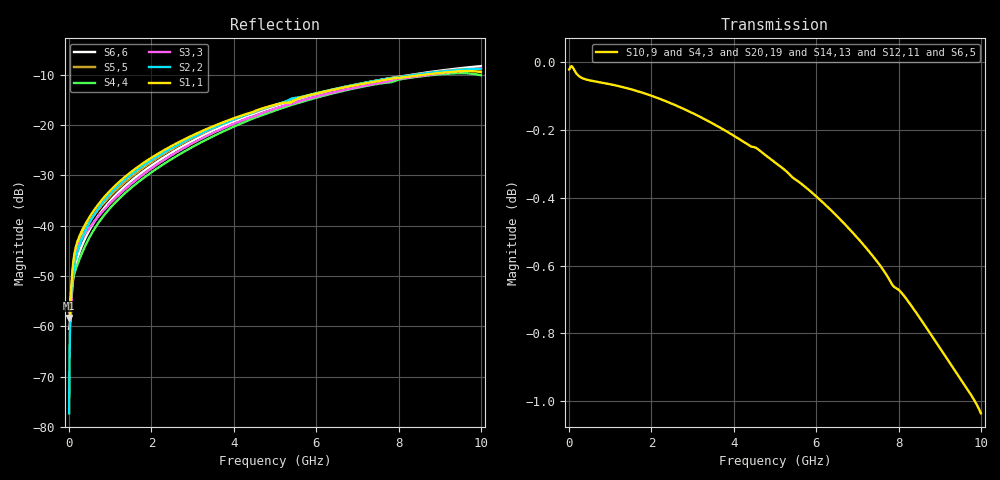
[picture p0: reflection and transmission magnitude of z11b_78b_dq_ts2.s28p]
![Disclaimer] This software code/ model/ data and all associated documentation, comments
!    or other information (collectively "Software") is provided
!    "AS IS" without warranty of any kind. MICRON TECHNOLOGY, INC.
!   ("MTI") EXPRESSLY DISCLAIMS ALL WARRANTIES EXPRESS OR IMPLIED,
!    INCLUDING BUT NOT LIMITED TO, NONINFRINGEMENT OF THIRD PARTY
!   RIGHTS, AND ANY IMPLIED WARRANTIES OF MERCHANTABILITY OR FITNESS
!    FOR ANY PARTICULAR PURPOSE. MTI DOES NOT WARRANT THAT THE
!    SOFTWARE WILL MEET YOUR REQUIREMENTS, OR THAT THE OPERATION OF
!    THE SOFTWARE WILL BE UNINTERRUPTED OR ERROR-FREE. FURTHERMORE,
!    MTI DOES NOT MAKE ANY REPRESENTATIONS REGARDING THE USE OR THE
!    RESULTS OF THE USE OF THE SOFTWARE IN TERMS OF ITS CORRECTNESS,
!    ACCURACY, RELIABILITY, OR OTHERWISE. THE ENTIRE RISK ARISING OUT
!    OF USE OR PERFORMANCE OF THE SOFTWARE REMAINS WITH YOU. IN NO
!    EVENT SHALL MTI, ITS AFFILIATED COMPANIES OR THEIR SUPPLIERS BE
!    LIABLE FOR ANY DIRECT, INDIRECT, CONSEQUENTIAL, INCIDENTAL, OR
!    SPECIAL DAMAGES (INCLUDING, WITHOUT LIMITATION, DAMAGES FOR LOSS
!    OF PROFITS, BUSINESS INTERRUPTION, OR LOSS OF INFORMATION)
!    ARISING OUT OF YOUR USE OF OR INABILITY TO USE THE SOFTWARE,
!    EVEN IF MTI HAS BEEN ADVISED OF THE POSSIBILITY OF SUCH DAMAGES.
!    Because some jurisdictions prohibit the exclusion or limitation
!    of liability for consequential or incidental damages, the above
!    limitation may not apply to you.
!    Copyright 2019 Micron Technology, Inc. All rights reserved.
! Single-ended  S-parameters
!NUMBER OF PORTS = 28
!  PORT#  PORT_NAME  NET_NAME
! PORT1:  DM#-BGA.A7 DM#
! PORT2:  DM#-Z11B_DIE.20 DM#
! PORT3:  DQ0-BGA.C2 DQ0
! PORT4:  DQ0-Z11B_DIE.26 DQ0
! PORT5:  DQ1-BGA.B7 DQ1
! PORT6:  DQ1-Z11B_DIE.22 DQ1
! PORT7:  DQ2-BGA.D3 DQ2
! PORT8:  DQ2-Z11B_DIE.28 DQ2
! PORT9:  DQ3-BGA.D7 DQ3
! PORT10:  DQ3-Z11B_DIE.24 DQ3
! PORT11:  DQ4-BGA.D2 DQ4
! PORT12:  DQ4-Z11B_DIE.37 DQ4
! PORT13:  DQ5-BGA.D8 DQ5
! PORT14:  DQ5-Z11B_DIE.33 DQ5
! PORT15:  DQ6-BGA.E3 DQ6
! PORT16:  DQ6-Z11B_DIE.39 DQ6
! PORT17:  DQ7-BGA.E7 DQ7
! PORT18:  DQ7-Z11B_DIE.35 DQ7
! PORT19:  DQS-C-BGA.B3 DQS-C
! PORT20:  DQS-C-Z11B_DIE.16 DQS-C
! PORT21:  DQS-T-BGA.C3 DQS-T
! PORT22:  DQS-T-Z11B_DIE.18 DQS-T
! PORT23:  VDD-VDD.BGA VDD
! PORT24:  VDD-VDD.Z11B_DIE VDD
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[Version] 2.0
# Hz S MA
[Number of Ports] 28
[Reference] 50 50 50 50 50 50 50 50 50 50 50 50 50 50 50 50 50 50 50 50 50 50 0.1 0.1 0.1 0.1 0.1 0.1
[Matrix Format] Full
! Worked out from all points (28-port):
!   1060 points, 10 Hz to 10 GHz, reference per port
!   strongest paths, dB at 10 Hz, 2.06 GHz, 4.71 GHz, 7.36 GHz, 10 GHz:
!     S10,9: 0.0, -0.1, -0.3, -0.6, -1.0
!     S4,3: 0.0, -0.1, -0.3, -0.6, -1.3
!     S20,19: 0.0, -0.1, -0.3, -0.5, -1.1
!     S14,13: 0.0, -0.1, -0.3, -0.6, -1.1
!     S12,11: 0.0, -0.1, -0.3, -0.6, -1.1
!     S6,5: 0.0, -0.1, -0.3, -0.6, -1.2
!   lowest |S11| = -58.4 dB at 10 Hz (marker M1), VSWR 1.00
!   |S11| at or under -10 dB: start of sweep to 8.615 GHz
